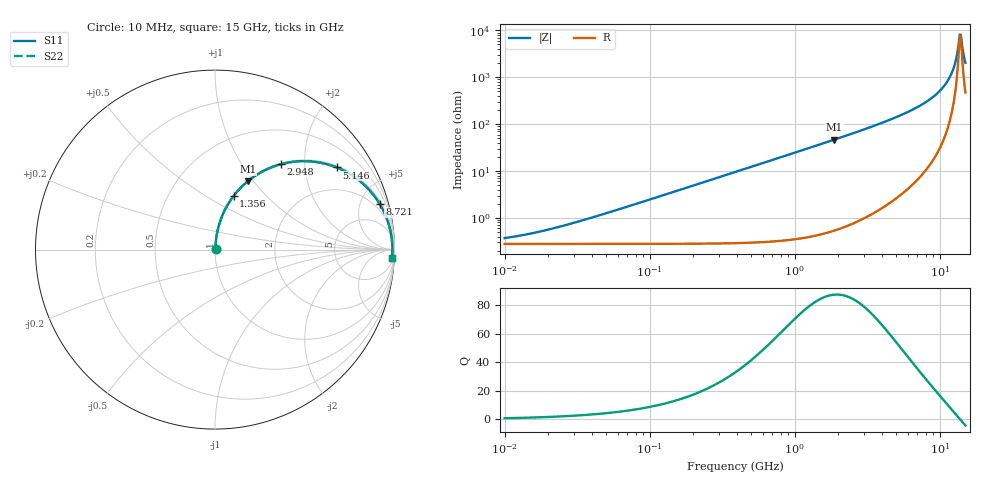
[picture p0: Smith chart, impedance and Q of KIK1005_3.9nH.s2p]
!version-3
!date-01.2023
!Series
# Hz S RI R 50
!Freq ReS11 ImS11 ReS21 ImS21 ReS12 ImS12 ReS22 ImS22
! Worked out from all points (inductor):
!   500 points, 10 MHz to 15 GHz, reference 50 ohm
!   read as one part in series: L = 3.9 nH near 34.25 MHz
!   highest Q = 87.1 at 1.872 GHz (marker M1), where L = 3.97 nH
!   self-resonance near 13.74 GHz
!   S11 on the Smith chart (normalised r, x): 10 MHz: 1.01, +0.00; 1.356 GHz: 1.01, +0.67; 2.948 GHz: 1.02, +1.51; 5.146 GHz: 1.06, +2.93; 8.721 GHz: 1.30, +7.08; 15 GHz: 10, -39
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1e7  0.00279 0.00244  0.9972 -0.00244  0.9972 -0.00244  0.00279 0.00244
1.745286e7  0.0028 0.00425  0.9972 -0.00425  0.9972 -0.00425  0.0028 0.00425
3.424937e7  0.00285 0.00834  0.9971 -0.00834  0.9971 -0.00834  0.00285 0.00834
1.155953e8  0.00359 0.0281  0.9964 -0.0281  0.9964 -0.0281  0.00359 0.0281
3.901468e8  0.0119 0.0943  0.9881 -0.0943  0.9881 -0.0943  0.0119 0.0943
1.316788e9  0.0988 0.2922  0.9012 -0.2922  0.9012 -0.2922  0.0988 0.2922
1.355956e9  0.1041 0.2993  0.8959 -0.2993  0.8959 -0.2993  0.1041 0.2993
1.871861e9  0.182 0.3801  0.818 -0.3801  0.818 -0.3801  0.182 0.3801
2.948397e9  0.3658 0.4754  0.6342 -0.4754  0.6342 -0.4754  0.3658 0.4754
4.444302e9  0.5943 0.4828  0.4057 -0.4828  0.4057 -0.4828  0.5943 0.4828
5.145797e9  0.6785 0.4576  0.3215 -0.4576  0.3215 -0.4576  0.6785 0.4576
6.89844e9  0.8282 0.3636  0.1718 -0.3636  0.1718 -0.3636  0.8282 0.3636
8.721466e9  0.9171 0.2555  0.0829 -0.2555  0.0829 -0.2555  0.9171 0.2555
1.039845e10  0.9611 0.1621  0.0389 -0.1621  0.0389 -0.1621  0.9611 0.1621
1.169197e10  0.979 0.0964  0.021 -0.0964  0.021 -0.0964  0.979 0.0964
1.258092e10  0.9855 0.0546  0.0145 -0.0546  0.0145 -0.0546  0.9855 0.0546
1.295514e10  0.9871 0.0377  0.0129 -0.0377  0.0129 -0.0377  0.9871 0.0377
1.353745e10  0.9884 0.0124  0.0116 -0.0124  0.0116 -0.0124  0.9884 0.0124
1.373731e10  0.9886 0.00397  0.0114 -0.00397  0.0114 -0.00397  0.9886 0.00397
1.414593e10  0.9884 -0.0129  0.0116 0.0129  0.0116 0.0129  0.9884 -0.0129
1.456671e10  0.9877 -0.0298  0.0123 0.0298  0.0123 0.0298  0.9877 -0.0298
1.5e10  0.9864 -0.0467  0.0136 0.0467  0.0136 0.0467  0.9864 -0.0467
